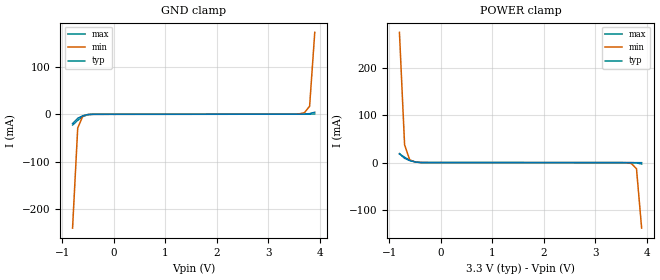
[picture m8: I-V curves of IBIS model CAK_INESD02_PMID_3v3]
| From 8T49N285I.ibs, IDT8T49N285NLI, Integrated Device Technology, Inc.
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| 4.00000e+00   -8.54915e-03   -4.17556e-01   -1.55019e-03
| 4.10000e+00   -1.91861e-02   -6.96800e-01   -7.03684e-03
| 4.20000e+00   -1.63453e-01   -9.76425e-01   -1.61732e-02
| 4.30000e+00   -5.37100e-01   -1.25631e+00   -2.57194e-02
| 4.40000e+00   -9.11109e-01   -1.53641e+00   -5.41179e-02
| 4.50000e+00   -1.28544e+00   -1.81670e+00   -4.53418e-01
| 4.60000e+00   -1.66006e+00   -2.09717e+00   -9.32246e-01
| 4.70000e+00   -2.03494e+00   -2.37780e+00   -1.41140e+00
| 4.80000e+00   -2.41006e+00   -2.65860e+00   -1.89082e+00
| 4.90000e+00   -2.78537e+00   -2.93955e+00   -2.37047e+00
| 5.00000e+00   -3.16087e+00   -3.22064e+00   -2.85029e+00
| 5.10000e+00   -3.53652e+00   -3.50186e+00   -3.33026e+00
| 5.20000e+00   -3.91230e+00   -3.78320e+00   -3.81034e+00
| 5.30000e+00   -4.28819e+00   -4.06466e+00   -4.29053e+00
| 5.40000e+00   -4.66418e+00   -4.34622e+00   -4.77081e+00
| 5.50000e+00   -5.04025e+00   -4.62788e+00   -5.25118e+00
| 5.60000e+00   -5.41640e+00   -4.90962e+00   -5.73160e+00
| 5.70000e+00   -5.79260e+00   -5.19145e+00   -6.21208e+00
| 5.80000e+00   -6.16885e+00   -5.47336e+00   -6.69259e+00
| 5.90000e+00   -6.54514e+00   -5.75534e+00   -7.17312e+00
| 6.00000e+00   -6.92147e+00   -6.03738e+00   -7.65366e+00
| 6.10000e+00   -7.29783e+00   -6.31948e+00   -8.13421e+00
| 6.20000e+00   -7.67421e+00   -6.60164e+00   -8.61476e+00
| 6.30000e+00   -8.05061e+00   -6.88385e+00   -9.09531e+00
| 6.40000e+00   -8.42702e+00   -7.16611e+00   -9.57585e+00
| 6.50000e+00   -8.80345e+00   -7.44841e+00   -1.00564e+01
| 6.60000e+00   -9.17988e+00   -7.73076e+00   -1.05369e+01
[Model] CAK_INESD02_PMID_3v3
Model_type   Input
Polarity   Non-Inverting
Vinl = 0.8V
Vinh = 2.0V
|   typ   min   max
C_comp   2pF   1.5pF   2.5pF
|   typ   min   max
[Voltage range]   3.3V   3.135V   3.465V
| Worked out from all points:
|   GND clamp passes 1 mA (typ) near -0.52 V on its own axis
|   POWER clamp passes 1 mA (typ) near -0.47 V on its own axis
[GND_clamp]
|Voltage   I (typ)   I (min)   I (max)
|Note, modeling breaks down at 250mA and above.  This is well beyond the functional   |
|operating range of the device.  Should this scenario occur, catastrophic failure and   |
|possible damage to the device and/or board is of higher concern than the I-V curve   |
|behavior.  The IBIS checker will flag currents in excess of 10A with warnings.  Lines   |
|with currents in excess of 0.35 A have been commented out.  The points still remain|
|available to the user if the user desires to use them.   |
|-3.30000e+00   -9.18001e+00   -7.26784e+00   -1.13299e+01
|-3.20000e+00   -8.80357e+00   -6.98557e+00   -1.08494e+01
|-3.10000e+00   -8.42715e+00   -6.70334e+00   -1.03689e+01
|-3.00000e+00   -8.05073e+00   -6.42116e+00   -9.88835e+00
|-2.90000e+00   -7.67433e+00   -6.13903e+00   -9.40781e+00
|-2.80000e+00   -7.29795e+00   -5.85697e+00   -8.92726e+00
|-2.70000e+00   -6.92159e+00   -5.57496e+00   -8.44671e+00
|-2.60000e+00   -6.54526e+00   -5.29303e+00   -7.96616e+00
|-2.50000e+00   -6.16897e+00   -5.01117e+00   -7.48561e+00
|-2.40000e+00   -5.79271e+00   -4.72939e+00   -7.00506e+00
|-2.30000e+00   -5.41651e+00   -4.44770e+00   -6.52454e+00
|-2.20000e+00   -5.04036e+00   -4.16610e+00   -6.04404e+00
|-2.10000e+00   -4.66429e+00   -3.88461e+00   -5.56358e+00
|-2.00000e+00   -4.28830e+00   -3.60322e+00   -5.08317e+00
|-1.90000e+00   -3.91240e+00   -3.32195e+00   -4.60283e+00
|-1.80000e+00   -3.53662e+00   -3.04081e+00   -4.12257e+00
|-1.70000e+00   -3.16097e+00   -2.75981e+00   -3.64242e+00
|-1.60000e+00   -2.78547e+00   -2.47896e+00   -3.16237e+00
|-1.50000e+00   -2.41015e+00   -2.19826e+00   -2.68245e+00
|-1.40000e+00   -2.03503e+00   -1.91773e+00   -2.20268e+00
|-1.30000e+00   -1.66015e+00   -1.63737e+00   -1.72311e+00
|-1.20000e+00   -1.28553e+00   -1.35720e+00   -1.24377e+00
|-1.10000e+00   -9.11197e-01   -1.07723e+00   -7.64721e-01
|-1.00000e+00   -5.37186e-01   -7.97502e-01   -2.86018e-01
|-9.00000e-01   -1.63537e-01   -5.18096e-01   -3.48489e-02
-800mV    -19.27mA   -239.2mA   -22.68mA
-700mV    -8.629mA   -28.98mA   -12.79mA
-600mV    -3.059mA   -3.709mA   -4.701mA
-500mV    -568.3uA   -621uA     -796.4uA
-400mV    -113.7uA   -126.5uA   -131.8uA
3.4V      69.72uA    69.11uA    76.75uA
3.6V      82.71uA    855.3uA    85.96uA
3.7V      215.4uA    3.374mA    90.69uA
3.8V      1.316mA    16.88mA    107.3uA
3.9V      4.218mA    172mA      475.4uA
| 4.00000e+00   9.04648e-03   4.59169e-01   2.66627e-03
| 4.10000e+00   1.91428e-02   7.45996e-01   7.17697e-03
| 4.20000e+00   1.92474e-01   1.03302e+00   1.38097e-02
| 4.30000e+00   5.75474e-01   1.32028e+00   2.02583e-02
| 4.40000e+00   9.58785e-01   1.60779e+00   5.15170e-02
| 4.50000e+00   1.34243e+00   1.89556e+00   4.81848e-01
| 4.60000e+00   1.72641e+00   2.18356e+00   9.72164e-01
| 4.70000e+00   2.11071e+00   2.47182e+00   1.46290e+00
| 4.80000e+00   2.49533e+00   2.76032e+00   1.95404e+00
| 4.90000e+00   2.88026e+00   3.04906e+00   2.44557e+00
| 5.00000e+00   3.26549e+00   3.33805e+00   2.93747e+00
| 5.10000e+00   3.65101e+00   3.62729e+00   3.42973e+00
| 5.20000e+00   4.03682e+00   3.91677e+00   3.92234e+00
| 5.30000e+00   4.42292e+00   4.20651e+00   4.41528e+00
| 5.40000e+00   4.80930e+00   4.49650e+00   4.90854e+00
| 5.50000e+00   5.19595e+00   4.78674e+00   5.40211e+00
| 5.60000e+00   5.58288e+00   5.07726e+00   5.89598e+00
| 5.70000e+00   5.97009e+00   5.36804e+00   6.39014e+00
| 5.80000e+00   6.35758e+00   5.65911e+00   6.88458e+00
| 5.90000e+00   6.74535e+00   5.95046e+00   7.37931e+00
| 6.00000e+00   7.13341e+00   6.24212e+00   7.87432e+00
| 6.10000e+00   7.52175e+00   6.53409e+00   8.36962e+00
| 6.20000e+00   7.91040e+00   6.82639e+00   8.86519e+00
| 6.30000e+00   8.29936e+00   7.11903e+00   9.36105e+00
| 6.40000e+00   8.68864e+00   7.41203e+00   9.85721e+00
| 6.50000e+00   9.07825e+00   7.70540e+00   1.03537e+01
| 6.60000e+00   9.46821e+00   7.99916e+00   1.08504e+01
[Power_clamp]
|Voltage   I (typ)   I (min)   I (max)
|Note, modeling breaks down at 250mA and above.  This is well beyond the functional   |
|operating range of the device.  Should this scenario occur, catastrophic failure and   |
|possible damage to the device and/or board is of higher concern than the I-V curve   |
|behavior.  The IBIS checker will flag currents in excess of 10A with warnings.  Lines   |
|with currents in excess of 0.35 A have been commented out.  The points still remain|
|available to the user if the user desires to use them.   |
|-3.30000e+00   9.46821e+00   7.51760e+00   1.16708e+01
|-3.20000e+00   9.07825e+00   7.22447e+00   1.11735e+01
|-3.10000e+00   8.68864e+00   6.93170e+00   1.06765e+01
|-3.00000e+00   8.29936e+00   6.63928e+00   1.01799e+01
|-2.90000e+00   7.91040e+00   6.34719e+00   9.68352e+00
|-2.80000e+00   7.52175e+00   6.05542e+00   9.18747e+00
|-2.70000e+00   7.13341e+00   5.76396e+00   8.69171e+00
|-2.60000e+00   6.74535e+00   5.47279e+00   8.19623e+00
|-2.50000e+00   6.35758e+00   5.18191e+00   7.70104e+00
|-2.40000e+00   5.97009e+00   4.89130e+00   7.20613e+00
|-2.30000e+00   5.58288e+00   4.60095e+00   6.71149e+00
|-2.20000e+00   5.19595e+00   4.31087e+00   6.21715e+00
|-2.10000e+00   4.80930e+00   4.02105e+00   5.72309e+00
|-2.00000e+00   4.42292e+00   3.73148e+00   5.22933e+00
|-1.90000e+00   4.03682e+00   3.44215e+00   4.73587e+00
|-1.80000e+00   3.65101e+00   3.15307e+00   4.24272e+00
|-1.70000e+00   3.26549e+00   2.86424e+00   3.74989e+00
|-1.60000e+00   2.88026e+00   2.57565e+00   3.25740e+00
|-1.50000e+00   2.49533e+00   2.28731e+00   2.76526e+00
|-1.40000e+00   2.11071e+00   1.99921e+00   2.27349e+00
|-1.30000e+00   1.72641e+00   1.71136e+00   1.78209e+00
|-1.20000e+00   1.34243e+00   1.42376e+00   1.29109e+00
|-1.10000e+00   9.58785e-01   1.13641e+00   8.00505e-01
|-1.00000e+00   5.75474e-01   8.49297e-01   3.10336e-01
|-9.00000e-01   1.92474e-01   5.62413e-01   2.81728e-02
-800mV    19.14mA    275.5mA    18.2mA
-700mV    9.046mA    37.66mA    11.3mA
-600mV    4.218mA    5.534mA    5.339mA
-500mV    1.316mA    1.453mA    1.631mA
-300mV    82.71uA    80.65uA    96.61uA
3.5V      -73.73uA   -91.03uA   -81.35uA
3.7V      -113.7uA   -1.953mA   -90.58uA
3.8V      -568.3uA   -12.92mA   -97.72uA
3.9V      -3.059mA   -138.7mA   -209.2uA
